FUNCTION_BLOCK FB_LN_IED_LD1_LEDGGIO1 EXTENDS FB_AcsiCommonLogicalNodeClass
VAR_INPUT
	NamPlt: FB_DO_IED_LD1_LEDGGIO1_NamPlt := (sClass:='LPL', bLinkResult:=THIS^.AddDataToContainer(ipData:=NamPlt));
	Beh: FB_DO_IED_LD1_LEDGGIO1_Beh := (sClass:='ENS', bLinkResult:=THIS^.AddDataToContainer(ipData:=Beh));
	Health: FB_DO_IED_LD1_LEDGGIO1_Health := (sClass:='ENS', bLinkResult:=THIS^.AddDataToContainer(ipData:=Health));
	Mod_: FB_DO_IED_LD1_LEDGGIO1_Mod := (sObjectName:='Mod', sClass:='ENC', bLinkResult:=THIS^.AddDataToContainer(ipData:=Mod_));
	SPCSO1: FB_DO_IED_LD1_LEDGGIO1_SPCSO1 := (sClass:='SPC', bLinkResult:=THIS^.AddDataToContainer(ipData:=SPCSO1));
END_VAR
VAR
END_VAR

END_FUNCTION_BLOCK
